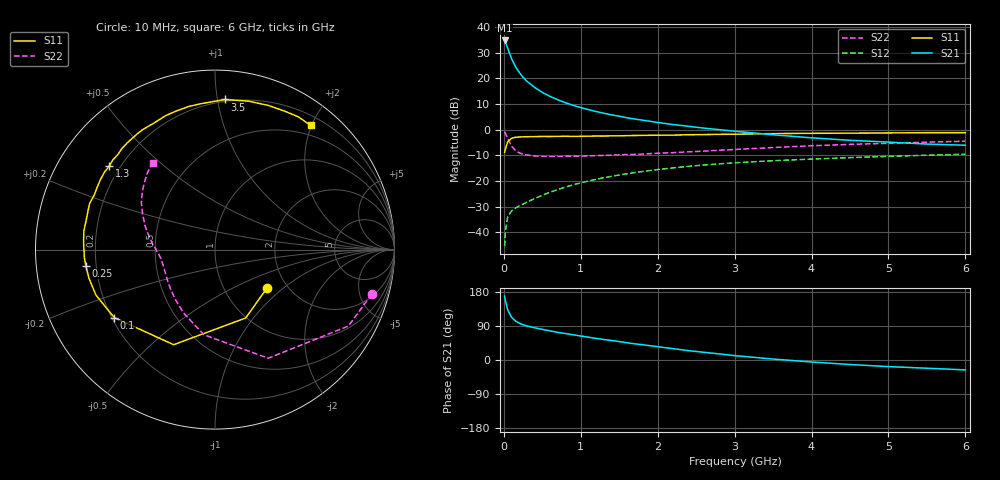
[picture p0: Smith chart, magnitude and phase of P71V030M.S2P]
! SIEMENS Small Signal Semiconductors
! BFP196
! Si NPN RF Bipolar Junction Transistor in SOT143
! VCE = 1 V  IC = 30 mA
! Common Emitter S-Parameters:  May  1996
# GHz  S  MA  R  50
!  f  S11  S21  S12  S22
! GHz  MAG  ANG  MAG  ANG  MAG  ANG  MAG  ANG
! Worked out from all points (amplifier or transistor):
!   36 points, 10 MHz to 6 GHz, reference 50 ohm
!   highest |S21| = 34.7 dB at 10 MHz (marker M1)
!   |S21| within 3 dB of that: start of sweep to 49.87 MHz
!   unconditionally stable (mu >= 1): 511.6 MHz to 5.444 GHz; 5.628 GHz to end of sweep
!   at 250 MHz: K = 0.75, MSG = 24.7 dB, |S12| = -29.0 dB
!   at 1.4 GHz: K = 1.11, MAG = 9.9 dB, |S12| = -18.2 dB
!   at 6 GHz: K = 1.00, MAG = 1.4 dB, |S12| = -9.6 dB
!   S11 on the Smith chart (normalised r, x): 10 MHz: 1.57, -0.78; 100 MHz: 0.21, -0.29; 250 MHz: 0.16, -0.06; 1.3 GHz: 0.16, +0.34; 3.5 GHz: 0.19, +1.05; 6 GHz: 0.34, +1.99
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0.01  0.3601 -37.0  54.48 168.5  0.0054 78.5  0.9085 -15.8
0.02  0.4176 -65.8  50.83 156.6  0.0105 71.3  0.8566 -29.8
0.05  0.5778 -113.5  38.52 132.7  0.0201 51.9  0.6742 -63.9
0.1  0.6773 -146.0  24.14 112.8  0.0261 42.4  0.4784 -97.4
0.15  0.7102 -159.1  16.98 103.1  0.0298 41.3  0.3943 -116.4
0.2  0.7199 -167.1  13.01 97.1  0.0329 42.0  0.3544 -128.7
0.25  0.7256 -172.9  10.46 93.0  0.0355 44.9  0.3321 -137.9
0.3  0.7291 -176.5  8.765 90.0  0.039 47.7  0.3212 -143.7
0.4  0.7334 176.8  6.641 85.1  0.0455 51.2  0.3085 -152.5
0.5  0.7379 171.9  5.313 80.9  0.0528 54.1  0.3031 -158.2
0.6  0.736 167.3  4.438 76.9  0.0605 55.7  0.3015 -162.1
0.7  0.7398 163.0  3.819 72.9  0.0681 56.5  0.3022 -165.1
0.9  0.7383 155.7  2.983 66.5  0.0844 56.4  0.3033 -169.6
1.1  0.7477 148.8  2.454 60.1  0.1002 55.6  0.3095 -172.8
1.3  0.751 141.6  2.088 54.0  0.1161 53.7  0.3151 -175.8
1.7  0.77 129.4  1.61 42.7  0.1461 49.3  0.3307 179.0
2.2  0.7829 115.7  1.256 30.0  0.1806 42.5  0.3568 172.8
2.8  0.8107 100.3  1 16.1  0.2161 34.0  0.3981 163.9
3.5  0.8382 86.2  0.795 2.5  0.2486 24.3  0.4488 154.0
4.5  0.8563 69.9  0.62 -11.9  0.2858 12.5  0.5169 141.6
5.5  0.8735 57.9  0.524 -21.7  0.3185 1.7  0.5715 131.0
6  0.873 52.4  0.498 -26.1  0.3328 -4.0  0.5967 125.7
